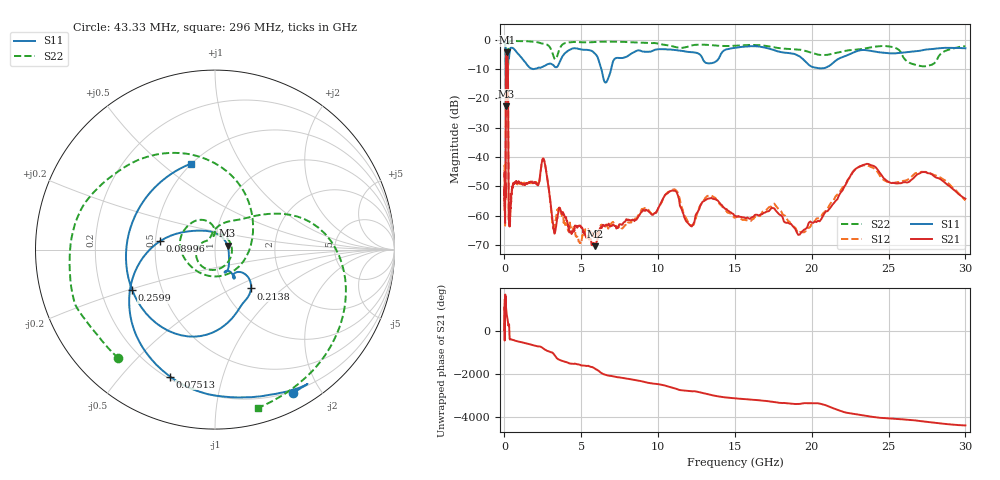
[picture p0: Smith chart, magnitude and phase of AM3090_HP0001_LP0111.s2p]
! Date/Time: Thu, Feb 28, 2019 1:54 PM
! Network Analyzer: Agilent Technologies E8364B Rev: A.07.50.67
! Sweep from 0.010 to 30.000 GHz, 1601 Points, Sweep Type: LOG
! Power Supply: 5.023 V, 0.002 A
# Hz S DB R 50
!freq MagS11 AngS11 MagS21 AngS21 MagS12 AngS12 MagS22 AngS22
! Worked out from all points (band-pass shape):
!   1601 points, 10 MHz to 30 GHz, reference 50 ohm
!   highest |S21| = -4.20 dB at 147.6 MHz (marker M1); lowest = -70.4 dB at 5.9 GHz (marker M2)
!   |S21| within 3 dB of the highest: 100.2 MHz to 216.6 MHz (116.4 MHz wide, 73.5 % of centre)
!   lowest |S11| = -22.7 dB at 98.44 MHz (marker M3), VSWR 1.16, Z = 57.5 + j2.45 ohm
!   |S11| at or under -10 dB: 89.84 MHz to 217.7 MHz (127.8 MHz wide, 83.1 % of centre); 6.309 GHz to 6.936 GHz (627.2 MHz wide, 9.47 % of centre)
!   |S22| runs from -23.8 to -0.2 dB; largest |S21 - S12| = 0.011
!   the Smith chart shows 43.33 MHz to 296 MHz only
!   S11 on the Smith chart (normalised r, x): 43.33 MHz: 0.18, -1.67; 75.13 MHz: 0.21, -0.69; 89.96 MHz: 0.53, +0.06; 213.8 MHz: 1.33, -0.63; 259.9 MHz: 0.34, -0.21; 296 MHz: 0.50, +0.63
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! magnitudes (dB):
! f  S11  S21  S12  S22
! 10 MHz  -0.3  -46.7  -46.8  -0.5
! 38.04 MHz  -0.5  -60.8  -58.7  -1.5
! 43.33 MHz  -0.8  -58.7  -61.9  -1.8
! 75.13 MHz  -2.5  -48.9  -46.1  -4.4
! 89.96 MHz  -10.2  -15.3  -15.3  -16.4
! 98.44 MHz  -22.7  -7.8  -7.8  -13.8
! 144.7 MHz  -15.1  -4.2  -4.2  -20.6
! 147.6 MHz  -15.1  -4.2  -4.2  -20.6
! 213.8 MHz  -10.6  -6.8  -6.7  -18.0
! 235.1 MHz  -7.9  -15.2  -15.2  -8.9
! 259.9 MHz  -5.8  -45.6  -45.2  -1.9
! 296 MHz  -6.1  -60.3  -63.1  -0.8
! 550.5 MHz  -2.8  -49.6  -49.5  -0.3
! 2.084 GHz  -9.8  -49.2  -48.7  -0.7
! 2.558 GHz  -9.0  -40.8  -40.7  -1.3
! 3.236 GHz  -8.9  -65.8  -63.7  -6.2
! 5.9 GHz  -4.7  -70.4  -66.9  -0.7
! 7.926 GHz  -5.8  -61.3  -62.8  -0.7
! 10.86 GHz  -3.3  -51.5  -51.4  -2.1
! 19.51 GHz  -7.0  -64.8  -65.7  -3.6
! 23.48 GHz  -3.5  -42.5  -42.9  -2.9
! 30 GHz  -2.8  -54.3  -54.8  -2.2
